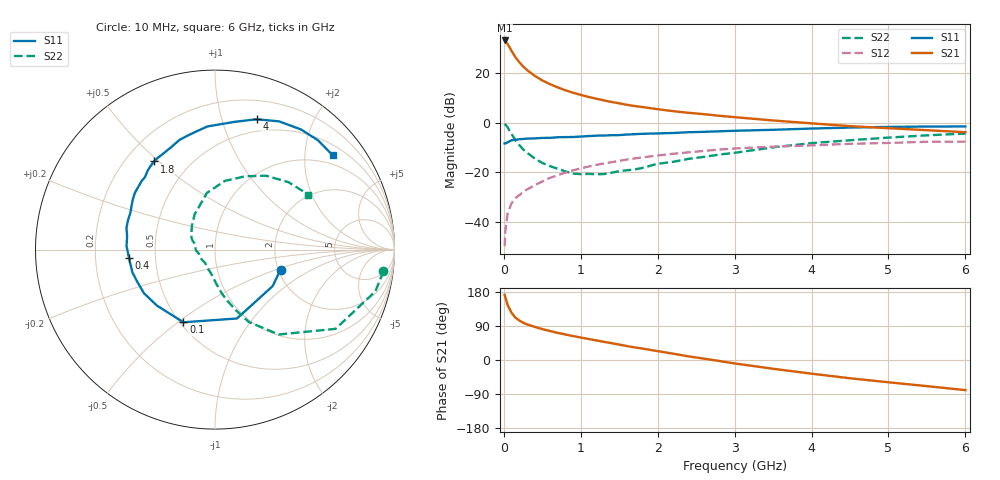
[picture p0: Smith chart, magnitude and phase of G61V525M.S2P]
! SIEMENS Small Signal Semiconductors
! BFG193
! Si NPN RF Bipolar Junction Transistor in SOT223
! VCE = 1.5 V  IC = 25 mA
! Common Emitter S-Parameters:  August  1996
# GHz  S  MA  R  50
!  f  S11  S21  S12  S22
! GHz  MAG  ANG  MAG  ANG  MAG  ANG  MAG  ANG
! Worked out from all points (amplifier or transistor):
!   36 points, 10 MHz to 6 GHz, reference 50 ohm
!   highest |S21| = 33.3 dB at 10 MHz (marker M1)
!   |S21| within 3 dB of that: start of sweep to 77.96 MHz
!   unconditionally stable (mu >= 1): 568.9 MHz to 2.7 GHz
!   at 250 MHz: K = 0.81, MSG = 25.4 dB, |S12| = -28.0 dB
!   at 1.4 GHz: K = 1.05, MAG = 10.7 dB, |S12| = -15.9 dB
!   at 6 GHz: K = 0.94, MSG = 1.9 dB, |S12| = -7.6 dB
!   S11 on the Smith chart (normalised r, x): 10 MHz: 2.06, -0.53; 100 MHz: 0.52, -0.52; 400 MHz: 0.35, -0.04; 1.8 GHz: 0.32, +0.48; 4 GHz: 0.37, +1.30; 6 GHz: 0.74, +2.66
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0.01  0.3819 -16.9  45.98 172.0  0.0032 85.2  0.9463 -7.3
0.02  0.3803 -32.3  44.68 164.9  0.0066 79.3  0.9232 -14.6
0.05  0.4028 -72.3  38.73 144.9  0.015 68.6  0.8039 -33.3
0.1  0.4416 -113.5  28.39 124.8  0.0235 61.1  0.5914 -53.1
0.15  0.4493 -136.0  21.16 111.8  0.0299 57.1  0.4458 -64.9
0.2  0.4646 -148.4  16.81 104.5  0.0343 57.7  0.356 -71.1
0.25  0.4692 -157.9  13.74 98.6  0.0396 58.4  0.2895 -76.8
0.3  0.4775 -164.7  11.67 94.2  0.0446 59.7  0.2496 -80.9
0.4  0.4817 -174.7  8.892 87.5  0.0545 60.8  0.1899 -88.0
0.5  0.4932 177.7  7.154 81.5  0.065 60.5  0.1537 -93.9
0.6  0.4953 171.4  6.021 76.4  0.0768 60.4  0.1329 -100.1
0.7  0.5082 166.1  5.183 71.6  0.0868 59.6  0.1175 -107.9
0.9  0.5144 156.3  4.04 63.2  0.1092 56.7  0.0937 -124.4
1.1  0.5374 148.3  3.323 55.5  0.1299 53.5  0.0923 -143.3
1.4  0.5591 137.1  2.624 44.4  0.1595 47.3  0.0975 -171.0
1.8  0.5973 124.7  2.075 30.3  0.1992 38.9  0.122 162.0
2.2  0.6206 113.2  1.714 16.7  0.2357 29.3  0.1619 144.1
3.5  0.7196 81.4  1.11 -23.1  0.3282 -2.2  0.3186 98.2
4  0.7624 72.3  0.971 -36.1  0.3483 -11.9  0.3868 81.8
4.5  0.7988 63.4  0.853 -48.2  0.3751 -21.8  0.4428 67.4
5.5  0.837 46.6  0.706 -69.0  0.4127 -44.5  0.5562 42.4
6  0.84 38.8  0.642 -79.5  0.4151 -57.4  0.6039 30.5
